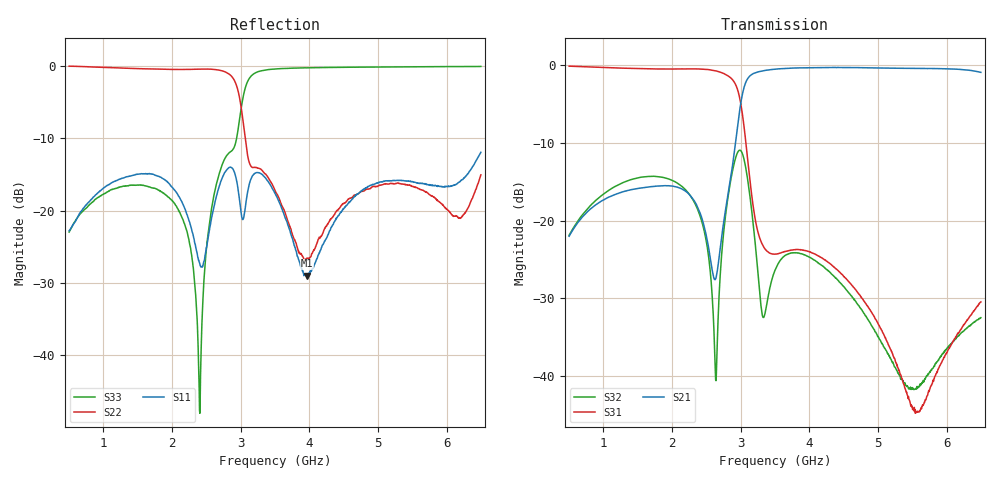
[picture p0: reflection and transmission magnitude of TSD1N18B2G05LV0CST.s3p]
# MHZ S RI R 50
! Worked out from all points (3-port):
!   1201 points, 500 MHz to 6.5 GHz, reference 50 ohm
!   strongest paths, dB at 500 MHz, 2 GHz, 3.5 GHz, 5 GHz, 6.5 GHz:
!     S21: -22.0, -15.6, -0.5, -0.3, -0.9
!     S31: -0.1, -0.5, -24.3, -33.3, -30.5
!     S32: -21.9, -14.8, -26.4, -34.9, -32.5
!   lowest |S11| = -29.0 dB at 3.965 GHz (marker M1), VSWR 1.07, Z = 52.1 + j2.94 ohm
!   |S11| at or under -10 dB: start of sweep to end of sweep
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500  -0.0314 -0.0653  0.0222 0.0759  0.9208 -0.3543
     0.0223 0.076  0.9096 -0.3988  0.0432 0.0679
     0.9219 -0.3522  0.0432 0.0678  -0.0196 -0.0683
2005  -0.1338 0.0536  0.1138 0.1217  -0.0424 -0.9453
      0.1143 0.1217  -0.1874 -0.9243  0.1033 -0.1492
      -0.0425 -0.9458  0.1031 -0.1489  -0.0967 -0.0643
2405  -0.0426 0.0026  0.0854 0.0737  -0.5257 -0.7879
      0.0852 0.0741  -0.5799 -0.7488  -0.0255 -0.105
      -0.5254 -0.7875  -0.0258 -0.105  0.00191 -0.00349
2640  -0.09 -0.0821  -0.0133 0.0409  -0.8043 -0.4488
      -0.0132 0.0405  -0.8117 -0.4744  -0.00524 0.0077
      -0.8032 -0.4488  -0.00507 0.00782  0.1472 -0.0122
2975  -0.00099 0.1269  -0.4613 0.1249  -0.4582 0.4553
      -0.4601 0.1241  -0.5286 0.342  0.074 -0.2721
      -0.4584 0.4549  0.074 -0.2728  0.3996 -0.00628
3320  -0.1678 -0.0538  -0.0291 0.9201  -0.0601 0.0352
      -0.0275 0.92  -0.1854 0.0266  0.00516 0.0236
      -0.06 0.0352  0.0051 0.0236  0.4455 -0.8127
3500  -0.1273 0.0316  0.2446 0.9115  -0.0608 -0.00307
      0.2445 0.9116  -0.1363 0.0193  0.0445 -0.0177
      -0.0607 -0.00326  0.0445 -0.0174  0.2118 -0.9254
3965  0.0215 0.0281  0.6545 0.7104  -0.0589 -0.0241
      0.654 0.7102  -0.027 -0.0385  0.0156 -0.0568
      -0.0589 -0.0245  0.0158 -0.0569  -0.1842 -0.9496
5550  0.0609 -0.1437  0.9514 -0.1024  -0.00187 0.00568
      0.9495 -0.1027  -0.0655 -0.1284  0.00379 -0.00738
      -0.00172 0.00568  0.00364 -0.00735  -0.7474 -0.6386
6500  0.2343 -0.0943  0.6299 -0.6423  0.0275 0.0122
      0.6317 -0.6424  0.0124 0.176  0.014 -0.0191
      0.0275 0.0119  0.0138 -0.0193  -0.8593 -0.4899
